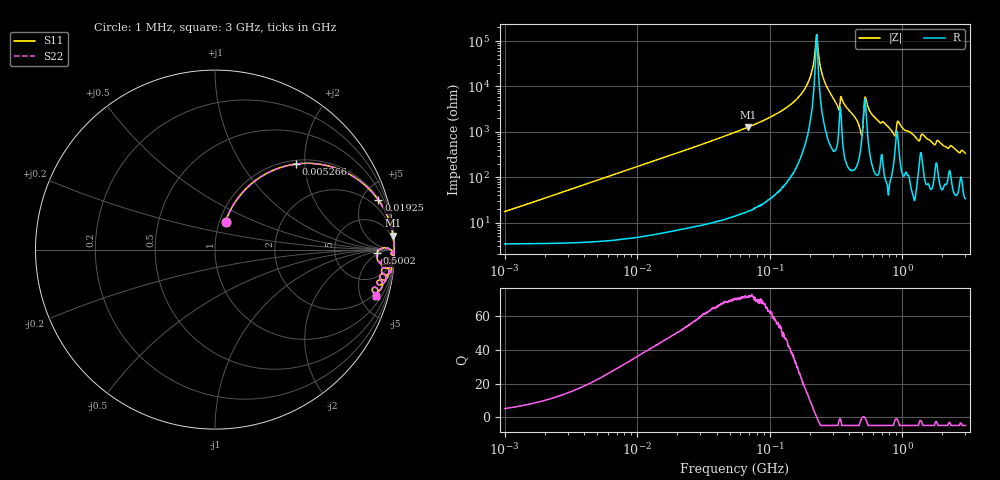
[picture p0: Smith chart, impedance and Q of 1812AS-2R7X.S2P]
!s-Parameter Generated by FASTRON Sdn. Bhd.
!FASTRON P/N : 1812AS-2R7X
!Keysight Technologies,E4991B,MY54100416,A.01.15
!Date created: Fri Oct 13 15:46:13 2023
!Version  : Rev00 Fri Oct 13 15:46:13 2023
!Data & Calibration Information:
!Freq	S11	S21	S12	S22
!PortZ  Port1:50+j0  Port2:50+j0
!When reading, reference impedance value at option line is always used.
! Remarks : This data is being provided solely for informational purposes.
# Hz S dB R 50
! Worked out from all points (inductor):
!   1601 points, 1 MHz to 3 GHz, reference 50 ohm
!   read as one part in series: L = 2.72 uH near 1.041 MHz
!   highest Q = 71.9 at 68.6 MHz (marker M1), where L = 2.93 uH
!   self-resonance near 225.7 MHz
!   S11 on the Smith chart (normalised r, x): 1 MHz: 1.07, +0.34; 5.266 MHz: 1.08, +1.80; 19.25 MHz: 1.13, +6.56; 500.2 MHz: 19, -4; 3 GHz: 1.67, -6.69
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1000000  -15.57 69.4  -0.41 -9.4  -0.41 -9.4  -15.57 69.4
3804036  -5.49 54.7  -1.75 -32.1  -1.75 -32.1  -5.49 54.7
5266264  -3.68 46.7  -2.75 -40.9  -2.75 -40.9  -3.68 46.7
1.447069e7  -0.73 21.9  -8.56 -66.8  -8.56 -66.8  -0.73 21.9
1.924694e7  -0.43 16.9  -10.75 -72.0  -10.75 -72.0  -0.43 16.9
5.477226e7  -0.06 5.8  -19.85 -83.3  -19.85 -83.3  -0.06 5.8
6.860483e7  -0.04 4.5  -22.08 -84.7  -22.08 -84.7  -0.04 4.5
1.520175e8  -0.01 1.3  -33.18 -87.1  -33.18 -87.1  -0.01 1.3
1.857042e8  -0.01 0.6  -39.30 -86.0  -39.30 -86.0  -0.01 0.6
2.083556e8  -0.01 0.3  -46.71 -81.9  -46.71 -81.9  -0.01 0.3
2.279937e8  -0.01 -0.0  -61.99 28.4  -61.99 28.4  -0.01 -0.0
2.558035e8  -0.01 -0.4  -43.14 83.0  -43.14 83.0  -0.01 -0.4
3.220132e8  -0.03 -1.4  -31.99 81.7  -31.99 81.7  -0.03 -1.4
3.541315e8  -0.03 -1.2  -33.84 80.9  -33.84 80.9  -0.03 -1.2
4.829509e8  -0.29 -4.8  -21.07 65.9  -21.07 65.9  -0.29 -4.8
5.001674e8  -0.88 -1.2  -20.12 11.0  -20.12 11.0  -0.88 -1.2
5.364635e8  -0.08 -1.0  -33.91 63.2  -33.91 63.2  -0.08 -1.0
7.925923e8  -0.05 -4.6  -21.95 83.2  -21.95 83.2  -0.05 -4.6
8.629671e8  -0.26 -6.1  -19.25 71.0  -19.25 71.0  -0.26 -6.1
9.490412e8  -0.14 -3.5  -24.01 73.6  -24.01 73.6  -0.14 -3.5
1.307284e9  -0.26 -8.2  -16.84 74.3  -16.84 74.3  -0.26 -8.2
3e9  -0.60 -16.0  -11.13 68.2  -11.13 68.2  -0.60 -16.0
